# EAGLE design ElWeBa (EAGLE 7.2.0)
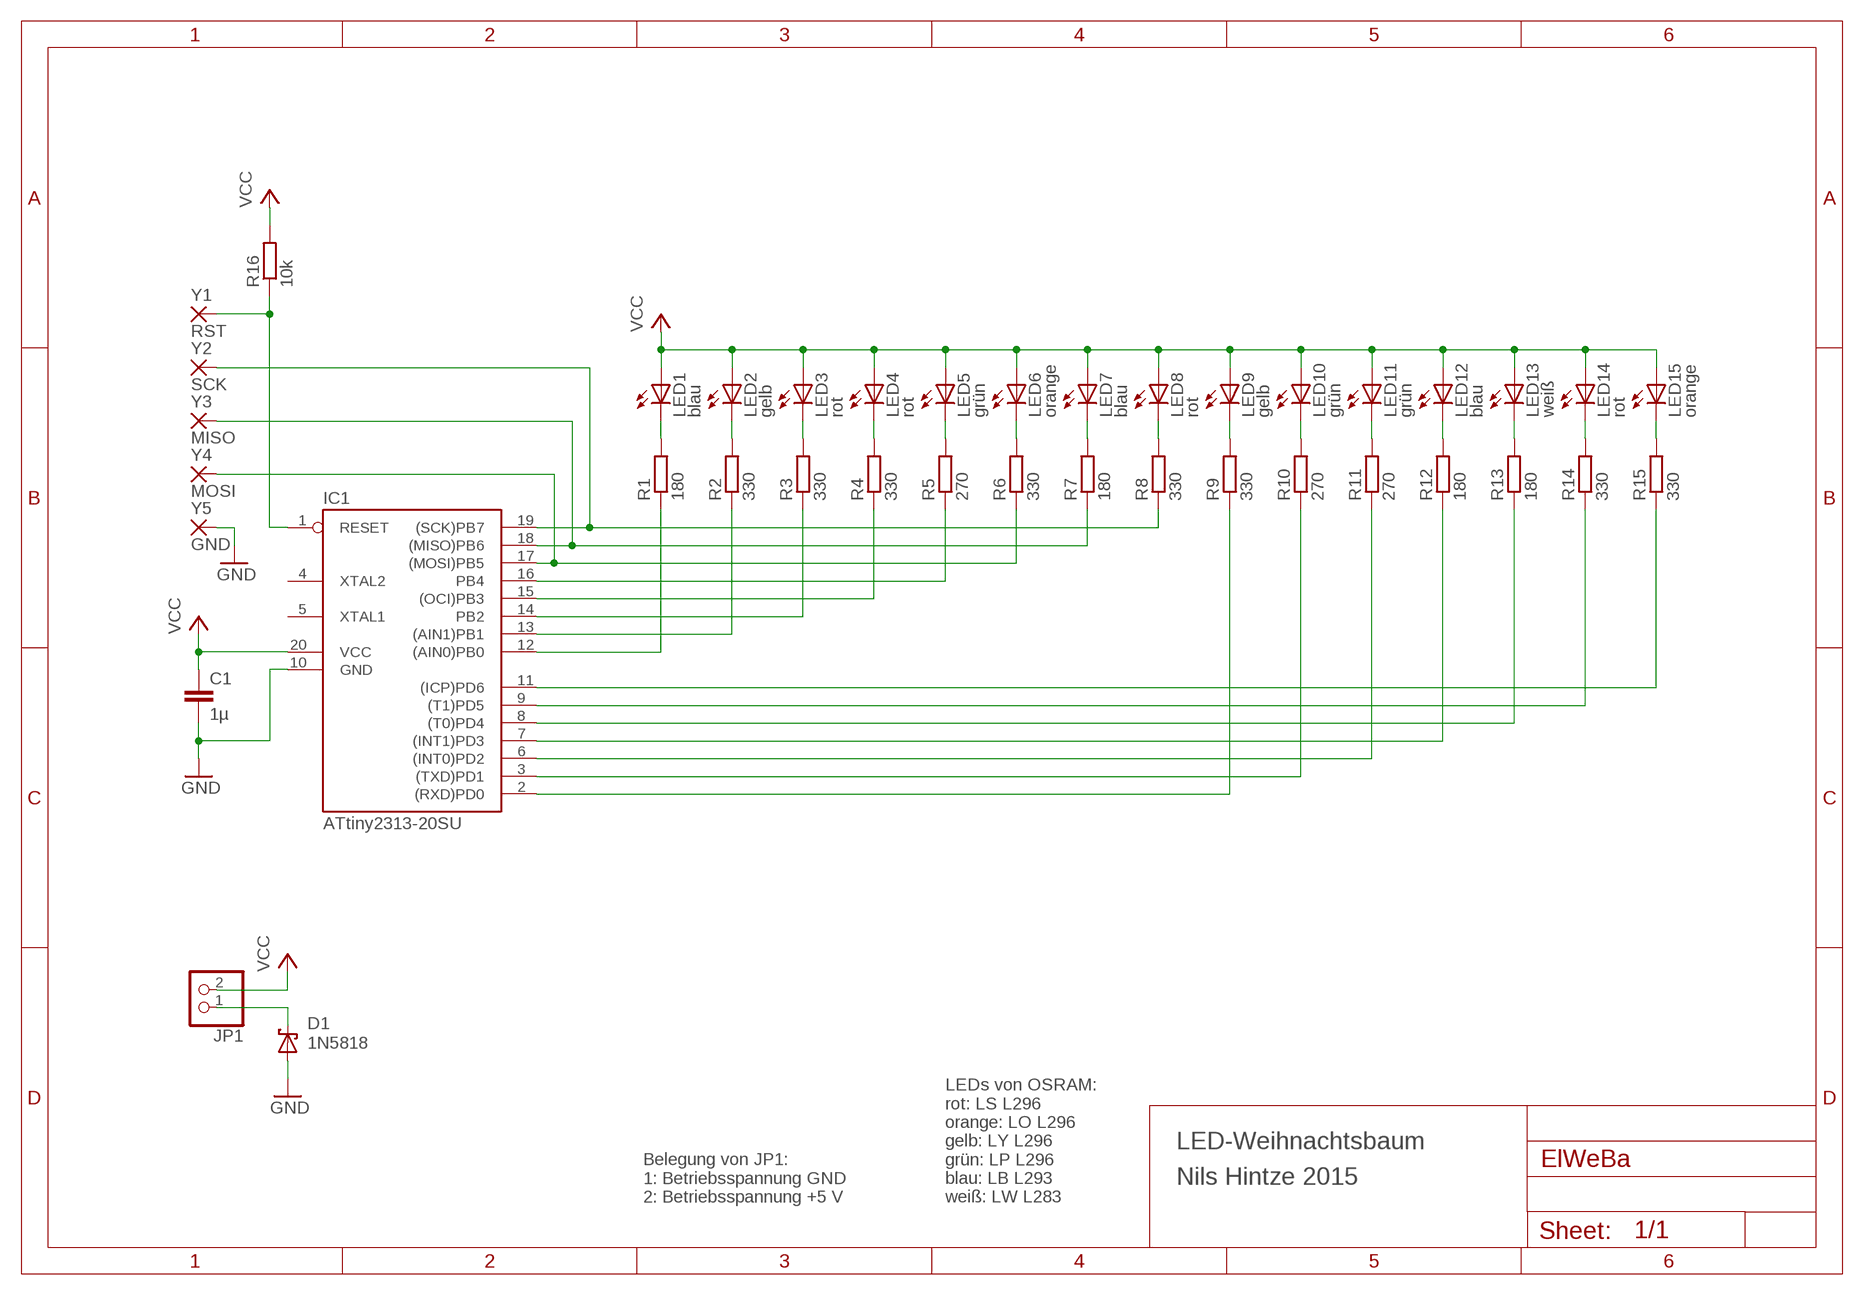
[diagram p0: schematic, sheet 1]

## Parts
C1  1µ  C-EUC1206  [C1206]
D1  1N5818  SCHOTTKY-DIODEDO41-17.5  [DO41-17.5]
IC1  ATtiny2313-20SU  AT90S2313S  [SO20L]
JP1  PINHD-1X2/90  [1X02/90]
LED1  blau  LEDCHIP-LED0805_LARGEPADS  [CHIP-LED0805_LARGEPADS]
LED2  gelb  LEDCHIP-LED0805_LARGEPADS  [CHIP-LED0805_LARGEPADS]
LED3  rot  LEDCHIP-LED0805_LARGEPADS  [CHIP-LED0805_LARGEPADS]
LED4  rot  LEDCHIP-LED0805_LARGEPADS  [CHIP-LED0805_LARGEPADS]
LED5  grün  LEDCHIP-LED0805_LARGEPADS  [CHIP-LED0805_LARGEPADS]
LED6  orange  LEDCHIP-LED0805_LARGEPADS  [CHIP-LED0805_LARGEPADS]
LED7  blau  LEDCHIP-LED0805_LARGEPADS  [CHIP-LED0805_LARGEPADS]
LED8  rot  LEDCHIP-LED0805_LARGEPADS  [CHIP-LED0805_LARGEPADS]
LED9  gelb  LEDCHIP-LED0805_LARGEPADS  [CHIP-LED0805_LARGEPADS]
LED10  grün  LEDCHIP-LED0805_LARGEPADS  [CHIP-LED0805_LARGEPADS]
LED11  grün  LEDCHIP-LED0805_LARGEPADS  [CHIP-LED0805_LARGEPADS]
LED12  blau  LEDCHIP-LED0805_LARGEPADS  [CHIP-LED0805_LARGEPADS]
LED13  weiß  LEDCHIP-LED0805_LARGEPADS  [CHIP-LED0805_LARGEPADS]
LED14  rot  LEDCHIP-LED0805_LARGEPADS  [CHIP-LED0805_LARGEPADS]
LED15  orange  LEDCHIP-LED0805_LARGEPADS  [CHIP-LED0805_LARGEPADS]
R1  180  R-EU_R0805  [R0805]
R2  330  R-EU_R0805  [R0805]
R3  330  R-EU_R0805  [R0805]
R4  330  R-EU_R0805  [R0805]
R5  270  R-EU_R0805  [R0805]
R6  330  R-EU_R0805  [R0805]
R7  180  R-EU_R0805  [R0805]
R8  330  R-EU_R0805  [R0805]
R9  330  R-EU_R0805  [R0805]
R10  270  R-EU_R0805  [R0805]
R11  270  R-EU_R0805  [R0805]
R12  180  R-EU_R0805  [R0805]
R13  180  R-EU_R0805  [R0805]
R14  330  R-EU_R0805  [R0805]
R15  330  R-EU_R0805  [R0805]
R16  10k  R-EU_R0805  [R0805]
Y1  RST  SMD5  [SMD2,54-5,08]
Y2  SCK  SMD5  [SMD2,54-5,08]
Y3  MISO  SMD5  [SMD2,54-5,08]
Y4  MOSI  SMD5  [SMD2,54-5,08]
Y5  GND  SMD5  [SMD2,54-5,08]

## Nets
GND: C1.2 D1.A IC1.10(GND) Y5.1(P)
N$1: LED1.C R1.2
N$2: LED2.C R2.2
N$3: LED3.C R3.2
N$4: LED4.C R4.2
N$5: LED5.C R5.2
N$6: LED6.C R6.2
N$7: LED7.C R7.2
N$8: IC1.12((AIN0)PB0) R1.1
N$9: IC1.13((AIN1)PB1) R2.1
N$10: IC1.14(PB2) R3.1
N$11: IC1.15((OCI)PB3) R4.1
N$12: IC1.16(PB4) R5.1
N$13: IC1.17((MOSI)PB5) R6.1 Y4.1(P)
N$14: IC1.18((MISO)PB6) R7.1 Y3.1(P)
N$15: IC1.19((SCK)PB7) R8.1 Y2.1(P)
N$16: IC1.2((RXD)PD0) R9.1
N$17: IC1.3((TXD)PD1) R10.1
N$18: IC1.6((INT0)PD2) R11.1
N$19: IC1.7((INT1)PD3) R12.1
N$20: IC1.8((T0)PD4) R13.1
N$21: IC1.9((T1)PD5) R14.1
N$22: IC1.11((ICP)PD6) R15.1
N$23: LED8.C R8.2
N$24: LED9.C R9.2
N$25: LED10.C R10.2
N$26: LED11.C R11.2
N$27: LED12.C R12.2
N$28: LED13.C R13.2
N$29: LED14.C R14.2
N$30: LED15.C R15.2
N$31: IC1.1(RESET) R16.1 Y1.1(P)
N$32: D1.C JP1.1
VCC: C1.1 IC1.20(VCC) JP1.2 LED1.A LED2.A LED3.A LED4.A LED5.A LED6.A LED7.A LED8.A LED9.A LED10.A LED11.A LED12.A LED13.A LED14.A LED15.A R16.2
Unconnected: IC1.4(XTAL2) IC1.5(XTAL1)

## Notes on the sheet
- LED-Weihnachtsbaum
- Nils Hintze 2015
- Belegung von JP1:
  1: Betriebsspannung GND
  2: Betriebsspannung +5 V
- LEDs von OSRAM:
  rot: LS L296
  orange: LO L296
  gelb: LY L296
  grün: LP L296
  blau: LB L293
  weiß: LW L283

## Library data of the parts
C1 = rcl:C-EU: CAPACITOR, European symbol
D1 = nh_diode:SCHOTTKY-DIODE: Schottky Diode
IC1 = atmel:AT90S2313: MICROCONTROLLER 2 Kbytes FLASH 128 bytes SRAM 128 bytes EEPROM UART; OC_FARNELL: unknown; OC_NEWARK: unknown
JP1 = pinhead:PINHD-1X2: PIN HEADER
LED1-LED15 = nh_led:LED: LED
R1-R16 = rcl:R-EU_: RESISTOR, European symbol
Y1-Y5 = wirepad:SMD5: SMD PAD

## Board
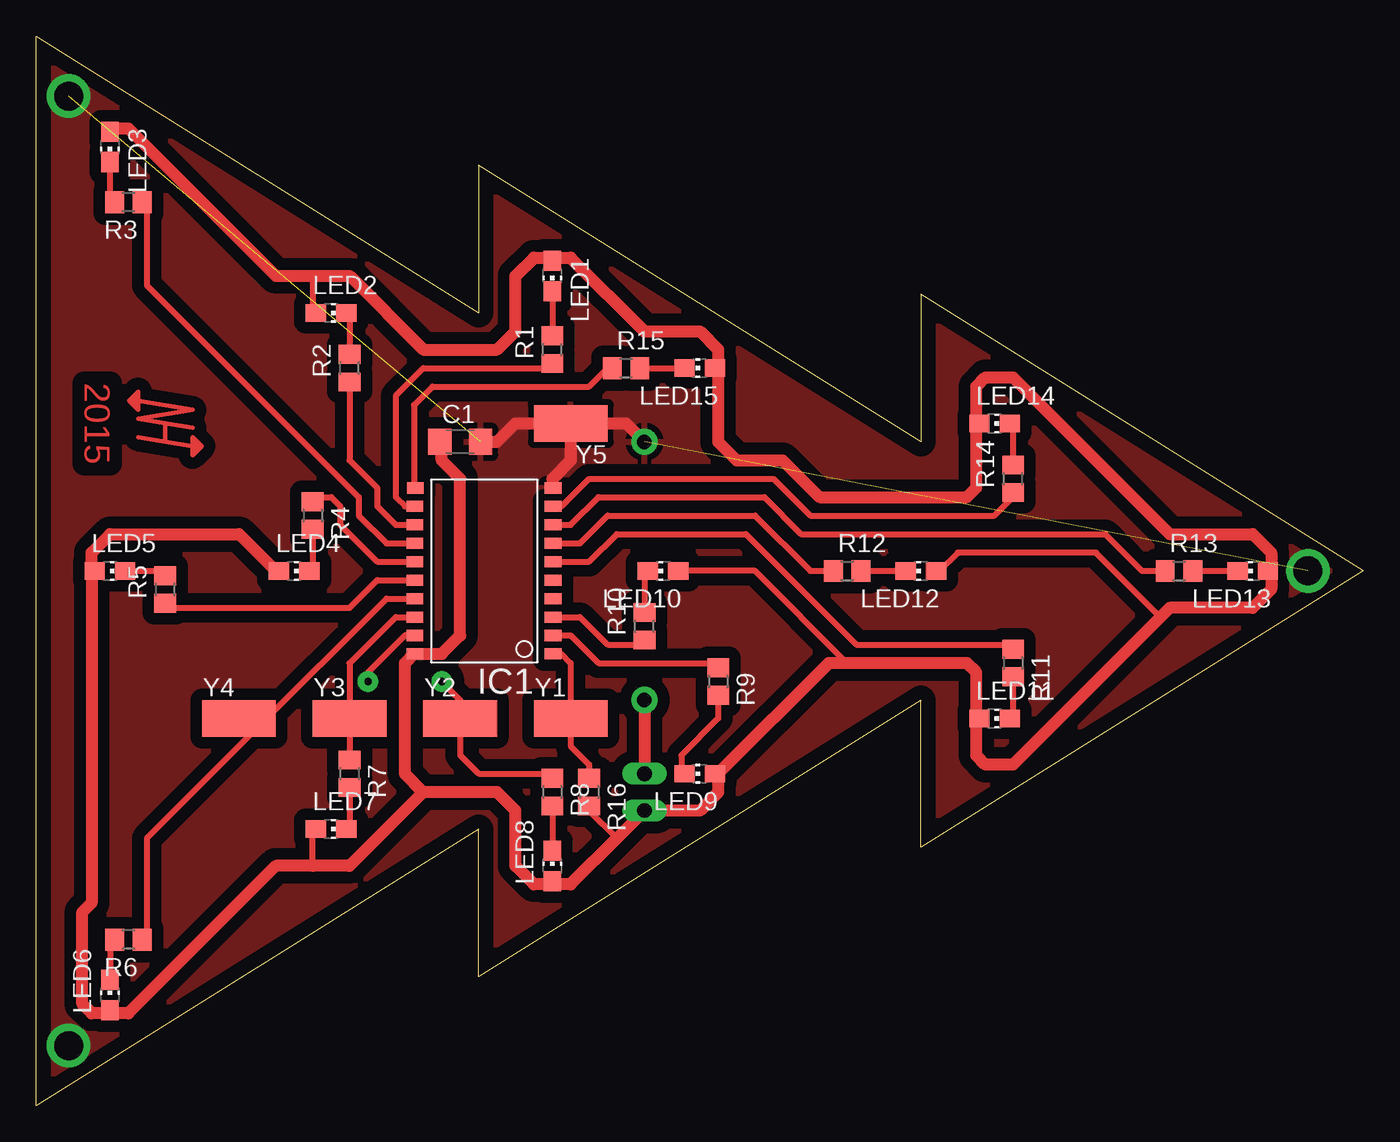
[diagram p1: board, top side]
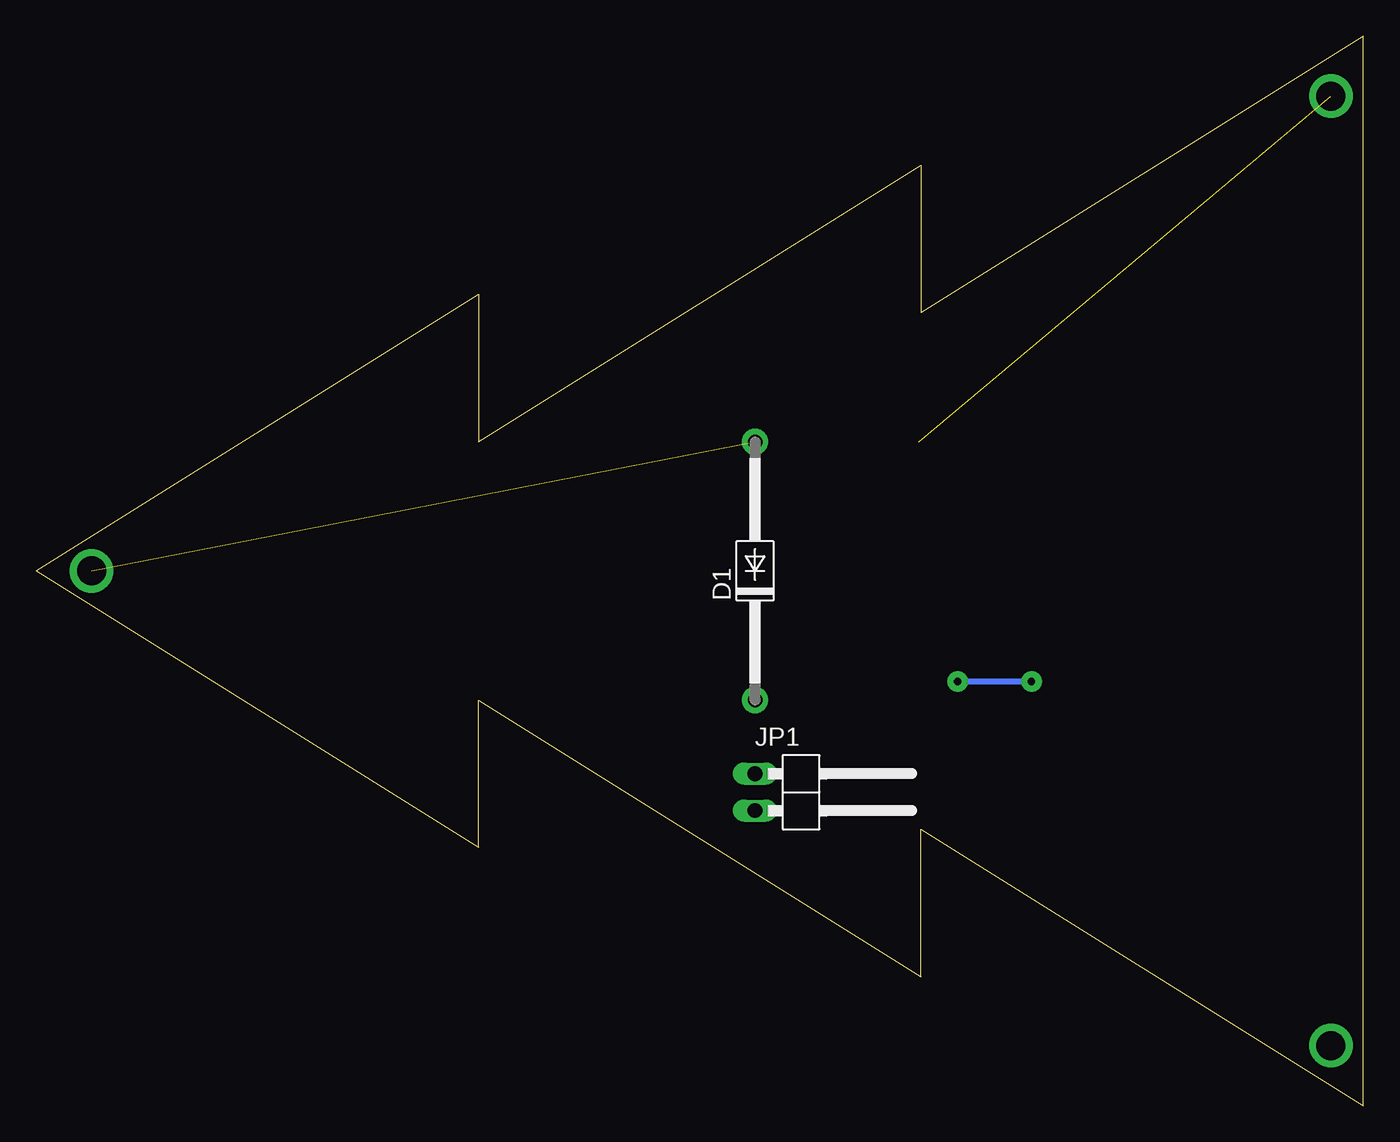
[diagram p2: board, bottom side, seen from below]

Size 91.44 x 73.66 mm. Coordinates in mm from the lower left corner, seen from the top.
Outline: 91.44,36.83 60.96,17.78 60.96,27.94 30.48,8.89 30.48,19.05 0,0 0,73.66 30.48,54.61 30.48,64.77 60.96,45.72 60.96,55.88 91.44,36.83
Copper layers (1*16): Top 0.035mm / dielectric 1.5mm / Bottom 0.035mm
Design rules "default *": minimum track width 10mil, minimum drill 24mil, track to track 8mil, track to pad 8mil, pad to pad 8mil, via to via 8mil, smd to smd 8mil, copper to edge 40mil, drill to drill 8mil, minimum pad ring 10mil, minimum via ring 8mil, stop-mask expansion 4mil, vias tented up to drill 0mil, thermal gap 16mil

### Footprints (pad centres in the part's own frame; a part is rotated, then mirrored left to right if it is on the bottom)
C1206 = smd 1.6 x 1.8: 1 -1.4,0; 2 1.4,0
DO41-17.5 = drill 1 pad 1.8: A 8.89,0; C -8.89,0
SO20L = smd 0.762 x 1.143: 1 -5.08,-5.131; 2 -3.81,-5.131; 3 -2.54,-5.131; 4 -1.27,-5.131; 5 0,-5.131; 6 1.27,-5.131; 7 2.54,-5.131; 8 3.81,-5.131; 9 5.08,-5.131; 10 6.35,-5.131; 11 6.35,4.369; 12 5.08,4.394; 13 3.81,4.394; 14 2.54,4.394; 15 1.27,4.394; 16 0,4.394; 17 -1.27,4.394; 18 -2.54,4.394; 19 -3.81,4.394; 20 -5.08,4.394
1X02/90 = drill 1.016 long: 1 -1.27,-3.81; 2 1.27,-3.81
CHIP-LED0805_LARGEPADS = smd 1.2 x 1.4: A 0,-1.05; C 0,1.05
R0805 = smd 1.3 x 1.5: 1 -0.95,0; 2 0.95,0
SMD2,54-5,08 = smd 2.54 x 5.08: 1 0,0

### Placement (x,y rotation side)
C1  29.21,45.72 0 top
D1  41.91,36.83 90 bottom
IC1  30.48,36.2 90 top
JP1  38.1,21.59 270 bottom
LED1  35.56,57.15 180 top
LED2  20.32,54.61 270 top
LED3  5.08,66.04 180 top
LED4  17.78,36.83 270 top
LED5  5.08,36.83 270 top
LED6  5.08,7.62 0 top
LED7  20.32,19.05 270 top
LED8  35.56,16.51 0 top
LED9  45.72,22.86 90 top
LED10  43.18,36.83 90 top
LED11  66.04,26.67 270 top
LED12  60.96,36.83 90 top
LED13  83.82,36.83 90 top
LED14  66.04,46.99 270 top
LED15  45.72,50.8 90 top
R1  35.56,52.07 90 top
R2  21.59,50.8 90 top
R3  6.35,62.23 180 top
R4  19.05,40.64 270 top
R5  8.89,35.56 90 top
R6  6.35,11.43 180 top
R7  21.59,22.86 270 top
R8  35.56,21.59 270 top
R9  46.99,29.21 270 top
R10  41.91,33.02 90 top
R11  67.31,30.48 270 top
R12  55.88,36.83 0 top
R13  78.74,36.83 0 top
R14  67.31,43.18 90 top
R15  40.64,50.8 0 top
R16  38.1,21.59 270 top
Y1  36.83,26.67 270 top
Y2  29.21,26.67 270 top
Y3  21.59,26.67 270 top
Y4  13.97,26.67 270 top
Y5  36.83,46.99 90 top

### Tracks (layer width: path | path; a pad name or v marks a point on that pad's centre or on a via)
GND  (via drill 2 pad 2.54)  (2 unrouted)
  Top 0.813: IC1.10 35.56,42.55 35.56,43.18 36.83,44.45 Y5.1 | C1.2 31.75,45.72 33.02,46.99 Y5.1 | Y5.1 40.64,46.99 D1.A
  other vias: 2.22,69.53 2.22,4.13 87.63,36.83
  pour Top (isolate 0.813): 0,0 30.48,19.05 30.48,8.89 60.96,27.94 60.96,17.78 91.44,36.83 60.96,55.88 60.96,45.72 30.48,64.77 30.48,54.61 0,73.66
N$1
  Top 0.406: LED1.C R1.2
N$2
  Top 0.406: LED2.C 21.59,54.61 R2.2
N$3
  Top 0.406: R3.2 5.08,62.23 LED3.C
N$4
  Top 0.406: LED4.C 19.05,36.83 R4.2
N$5
  Top 0.406: R5.2 8.89,36.83 LED5.C
N$6
  Top 0.406: R6.2 5.08,11.43 LED6.C
N$7
  Top 0.406: LED7.C 21.59,19.05 R7.2
N$8
  Top 0.406: IC1.12 25.4,41.27 24.77,41.91 24.77,48.9 26.67,50.8 35.56,50.8 R1.1
N$9
  Top 0.406: R2.1 21.59,44.45 23.5,42.55 23.5,41.27 24.77,40.01 IC1.13
N$10
  Top 0.406: R3.1 7.62,62.23 7.62,56.52 22.23,41.91 22.23,40.64 24.13,38.73 IC1.14
N$11
  Top 0.406: R4.1 19.05,41.91 20.32,41.91 20.95,41.27 20.95,40.01 23.5,37.47 IC1.15
N$12
  Top 0.406: R5.1 8.89,34.29 21.59,34.29 23.5,36.2 IC1.16
N$13
  Top 0.406: R6.1 7.62,11.43 7.62,18.41 14.92,25.72 | 14.92,25.72 24.13,34.92 IC1.17 | Y4.1 14.92,25.72
N$14
  Top 0.406: IC1.18 24.77,33.66 21.59,30.48 Y3.1 R7.1
N$15  (via drill 0.5 pad 1.42)
  Top 0.406: R8.1 35.56,22.86 30.48,22.86 29.21,24.13 Y2.1 29.21,27.94 v27.94,29.21 | v22.86,29.21 22.86,29.84 25.4,32.38 IC1.19
  Bottom 0.406: v22.86,29.21 v27.94,29.21
N$16
  Top 0.406: IC1.2 36.83,32.38 38.73,30.48 46.99,30.48 R9.1
N$17
  Top 0.406: R10.1 41.91,31.75 39.37,31.75 37.47,33.66 IC1.3
N$18
  Top 0.406: IC1.6 38.1,37.47 40.01,39.37 48.9,39.37 56.52,31.75 67.31,31.75 R11.1
N$19
  Top 0.406: IC1.7 37.47,38.73 39.37,40.64 49.53,40.64 53.34,36.83 R12.1
N$20
  Top 0.406: IC1.8 36.83,40.01 38.73,41.91 50.16,41.91 52.7,39.37 73.66,39.37 76.2,36.83 R13.1
N$21
  Top 0.406: IC1.9 36.2,41.27 38.1,43.18 50.8,43.18 53.34,40.64 66.04,40.64 67.31,41.91 R14.1
N$22
  Top 0.406: R15.1 39.37,50.8 38.1,49.53 27.3,49.53 26.04,48.26 26.04,42.55 IC1.11
N$23
  Top 0.406: R8.2 LED8.C
N$24
  Top 0.406: R9.2 46.99,26.67 44.45,24.13 44.45,22.86 LED9.C
N$25
  Top 0.406: LED10.C 41.91,36.83 R10.2
N$26
  Top 0.406: LED11.C 67.31,26.67 R11.2
N$27
  Top 0.406: R12.2 LED12.C
N$28
  Top 0.406: R13.2 LED13.C
N$29
  Top 0.406: LED14.C 67.31,46.99 R14.2
N$30
  Top 0.406: R15.2 LED15.C
N$31
  Top 0.406: IC1.1 36.2,31.11 36.83,30.48 Y1.1 36.83,24.77 38.1,23.5 R16.1
N$32
  Top 0.813: D1.C JP1.1
N$100
  Top 0.312: 7.01,48.55 10.77,47.93 7.01,47.3 8.89,46.99 | 8.89,46.99 10.77,46.68 | 8.89,46.99 8.89,45.74 | 7.01,46.05 8.89,45.74 | 8.89,45.74 10.77,45.43 | 7.01,48.55 7.01,49.18 6.7,48.87 | 7.01,48.55 7.01,47.93 6.7,48.24 | 6.7,48.24 6.39,48.55 6.7,48.87 | 6.7,48.24 6.7,48.87 | 11.08,45.74 10.77,46.05 10.77,45.43 | 11.08,45.74 11.39,45.43 11.08,45.12 | 11.08,45.12 10.77,44.8 10.77,45.43 | 11.08,45.74 11.08,45.12
VCC
  Top 0.406: LED2.A 19.05,54.61 19.05,57.15 | 35.56,58.42 LED1.A | 46.99,50.8 LED15.A | 64.77,46.99 LED14.A | 64.77,26.67 LED11.A | 5.08,6.35 LED6.A | 46.99,22.86 LED9.A | LED10.A 49.53,36.83 55.88,30.48 | LED12.A 62.23,36.83 63.5,38.1 73.03,38.1 77.47,33.66 | 19.05,16.51 19.05,19.05 LED7.A | 85.09,36.83 LED13.A | 35.56,15.24 LED8.A | R16.2 38.1,20.32 40.01,18.41 | LED5.A 3.81,36.83
  Top 0.813: LED3.A 5.08,67.31 6.35,67.31 16.51,57.15 19.05,57.15 21.59,57.15 26.67,52.07 31.75,52.07 33.02,53.34 33.02,57.15 34.29,58.42 35.56,58.42 36.83,58.42 41.91,53.34 45.72,53.34 46.99,52.07 46.99,50.8 46.99,45.72 48.26,44.45 51.44,44.45 53.98,41.91 64.14,41.91 64.77,42.55 64.77,46.99 64.77,49.53 65.41,50.16 67.31,50.16 78.11,39.37 83.82,39.37 85.09,38.1 85.09,36.83 85.09,35.56 83.82,34.29 78.11,34.29 77.47,33.66 67.31,23.5 65.41,23.5 64.77,24.13 64.77,26.67 64.77,29.84 64.14,30.48 55.88,30.48 54.61,30.48 46.99,22.86 46.99,21.59 45.72,20.32 JP1.2 40.01,18.41 36.83,15.24 35.56,15.24 34.29,15.24 33.02,16.51 33.02,20.32 31.75,21.59 26.67,21.59 | LED4.A 16.51,36.83 13.97,39.37 5.08,39.37 3.81,38.1 3.81,36.83 3.81,13.97 3.17,13.34 3.17,6.99 3.81,6.35 5.08,6.35 6.35,6.35 16.51,16.51 19.05,16.51 21.59,16.51 26.67,21.59 | 26.67,21.59 25.4,22.86 25.4,30.48 26.04,31.11 IC1.20 27.94,31.11 29.21,32.38 29.21,43.18 27.94,44.45 27.94,45.72 C1.1

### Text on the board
Top: 2015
